(* Logix 5000 AddOnInstructionDefinition export Banner_LM_PD_v4; software revision 33.00 *)

TYPE Banner_LM_PDIO_v4 :   // UDT that records the converted prcoess data.
STRUCT
   Channel_1_Output_State : SINT;   // 0 = Inactive, 1 = Active
   Analog_State : SINT;   // 0 = Inactive, 1 = Active.
   Sensor_Stability : SINT;   // 0 = No target or Marginal signal, 1 = Stable signal
   Measurement_Value_1 : REAL;   // Measured distance in micrometers
   Measurement_Value_2 : REAL;   // Measured distance in micrometers
   Transducer_Disable : INT;   // 0 = Laser On, 1 = Laser Off.
   PDI_DT : SINT[4];
   PDO_DT : SINT[2];
END_STRUCT
END_TYPE

ADD_ON_INSTRUCTION Banner_LM_PD_v4   (* revision 4.0, vendor Banner Engineering *)
// Takes the raw SINT Process Data Input information and converts that data into actual information.  Sends Process Data Output information to sensor.
VAR_IN_OUT
   Process_Data : Banner_LM_PDIO_v4; {required}
END_VAR
VAR_INPUT
   Binary_Include : SINT; {required}   // Determines if binary data is included in the Proces data
   PD_Measurement_1 : SINT; {required}   // Measurment mode of the Sensor. Tells AOI how to format the data.
   PD_Measurement_2 : SINT; {required}   // Measurment mode of the Sensor. Tells AOI how to format the data.
   Byte_Swap : BOOL; {required}   // Swap the LSB and the MSB with each other.
END_VAR
VAR
   Temp_Measurement_1 : DINT; {access None}
   Data_Byte : SINT[4]; {access None}
   Temp_Measurement_2 : DINT; {access None}
END_VAR

ROUTINE Logic   (* ladder *)
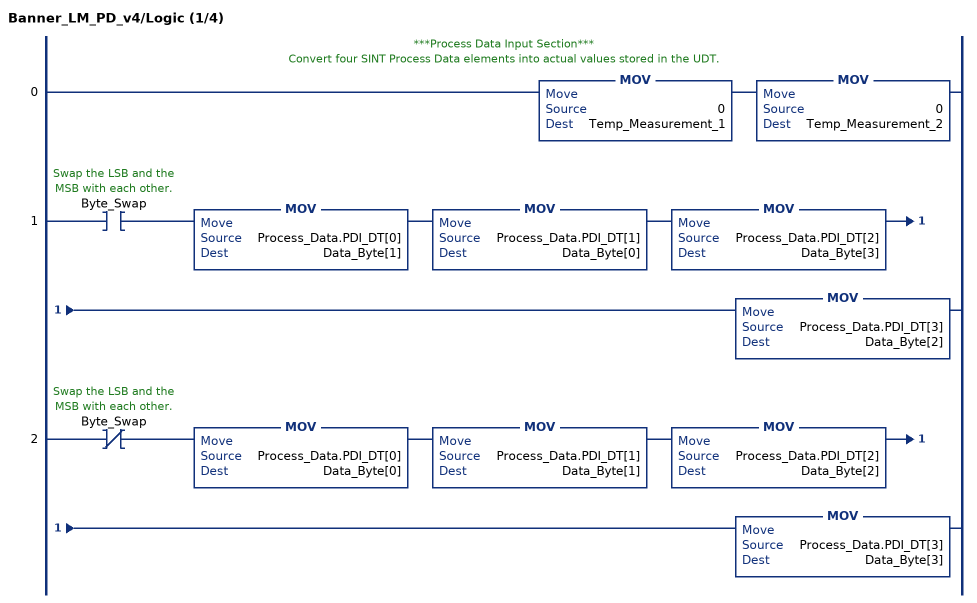
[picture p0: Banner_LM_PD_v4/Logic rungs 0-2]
   // ***Process Data Input Section***
   // Convert four SINT Process Data elements into actual values stored in the UDT.
   0: MOV(0,Temp_Measurement_1)MOV(0,Temp_Measurement_2);
   1: XIC(Byte_Swap)MOV(Process_Data.PDI_DT[0],Data_Byte[1])MOV(Process_Data.PDI_DT[1],Data_Byte[0])MOV(Process_Data.PDI_DT[2],Data_Byte[3])MOV(Process_Data.PDI_DT[3],Data_Byte[2]);
   2: XIO(Byte_Swap)MOV(Process_Data.PDI_DT[0],Data_Byte[0])MOV(Process_Data.PDI_DT[1],Data_Byte[1])MOV(Process_Data.PDI_DT[2],Data_Byte[2])MOV(Process_Data.PDI_DT[3],Data_Byte[3]);
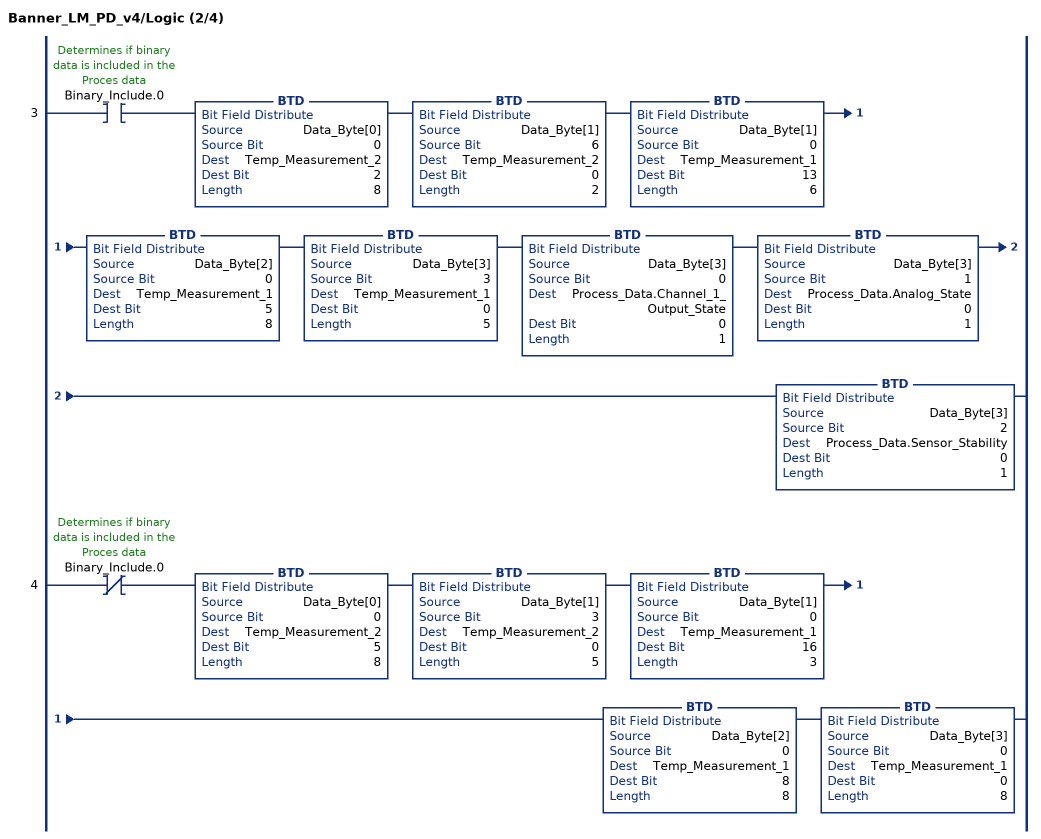
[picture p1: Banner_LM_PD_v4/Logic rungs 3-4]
   3: XIC(Binary_Include.0)BTD(Data_Byte[0],0,Temp_Measurement_2,2,8)BTD(Data_Byte[1],6,Temp_Measurement_2,0,2)BTD(Data_Byte[1],0,Temp_Measurement_1,13,6)BTD(Data_Byte[2],0,Temp_Measurement_1,5,8)BTD(Data_Byte[3],3,Temp_Measurement_1,0,5)BTD(Data_Byte[3],0,Process_Data.Channel_1_Output_State,0,1)BTD(Data_Byte[3],1,Process_Data.Analog_State,0,1)BTD(Data_Byte[3],2,Process_Data.Sensor_Stability,0,1);
   4: XIO(Binary_Include.0)BTD(Data_Byte[0],0,Temp_Measurement_2,5,8)BTD(Data_Byte[1],3,Temp_Measurement_2,0,5)BTD(Data_Byte[1],0,Temp_Measurement_1,16,3)BTD(Data_Byte[2],0,Temp_Measurement_1,8,8)BTD(Data_Byte[3],0,Temp_Measurement_1,0,8);
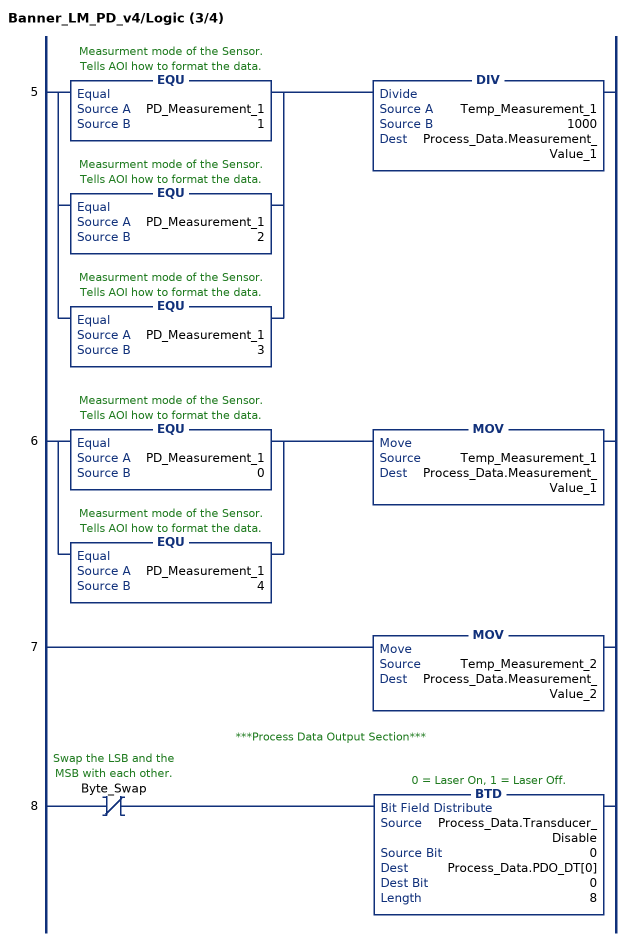
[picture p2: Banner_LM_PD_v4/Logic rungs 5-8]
   5: [EQU(PD_Measurement_1,1) ,EQU(PD_Measurement_1,2) ,EQU(PD_Measurement_1,3) ]DIV(Temp_Measurement_1,1000,Process_Data.Measurement_Value_1);
   6: [EQU(PD_Measurement_1,0) ,EQU(PD_Measurement_1,4) ]MOV(Temp_Measurement_1,Process_Data.Measurement_Value_1);
   7: MOV(Temp_Measurement_2,Process_Data.Measurement_Value_2);
   // ***Process Data Output Section***
   8: XIO(Byte_Swap)BTD(Process_Data.Transducer_Disable,0,Process_Data.PDO_DT[0],0,8);
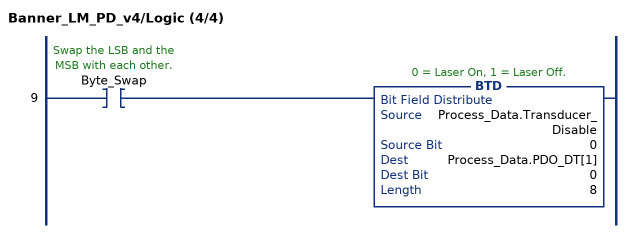
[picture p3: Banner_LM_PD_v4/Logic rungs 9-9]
   9: XIC(Byte_Swap)BTD(Process_Data.Transducer_Disable,0,Process_Data.PDO_DT[1],0,8);
END_ROUTINE
END_ADD_ON_INSTRUCTION
